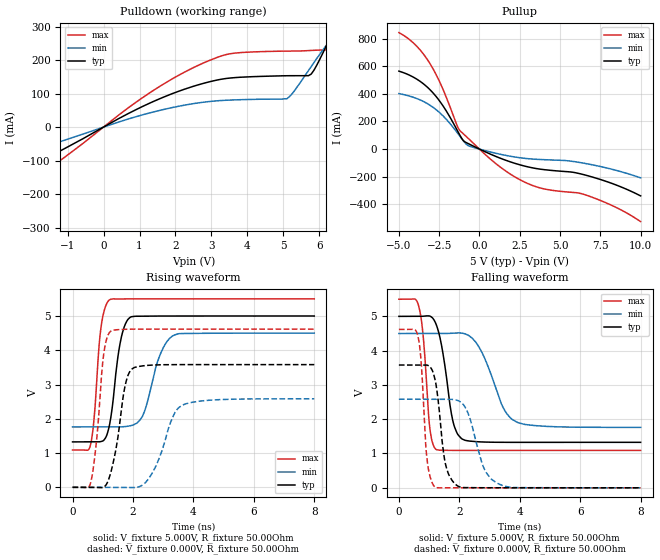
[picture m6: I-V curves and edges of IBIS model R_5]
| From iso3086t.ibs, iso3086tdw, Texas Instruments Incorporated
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|   R_5 MODEL
[Model]   R_5
Model_type   3-state
Polarity   Non-Inverting
Enable   Active-Low
Vmeas   = 2.5V
Vref   = 0V
Cref   = 15pF
|   typ   min   max
|Average C_comp   (Fast PVT)   (Nom PVT)   (Slow PVT)
C_comp   1.85212465pF 1.8517676pF  1.8666174pF
|C_comp (High state)   (Fast PVT)   (Nom PVT)   (Slow PVT)
|C_comp   1.9127669pF  1.9018070pF  1.9152375pF
|C_comp (Low state)   (Fast PVT)   (Nom PVT)   (Slow PVT)
|C_comp   1.7890118pF  1.8017282pF  1.8204679pF
[Model Spec]
Vmeas   2.5V   2.25V   2.75V
[Voltage Range]   5   4.5   5.5
[Temperature Range]   40   125   -40
[Pullup Reference]   5   4.5   5.5
[Pulldown Reference]   0   0   0
[Power Clamp Reference]   5   4.5   5.5
[GND Clamp Reference]   0   0   0
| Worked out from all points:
|   slope of the pulldown table from 0 to 0.75 V, typ, clamps not added: 17.1 ohm
|   slope of the pullup table from 0 to 0.75 V, typ, clamps not added: 18.8 ohm
|   falling waveform, V_fixture 5.000V, R_fixture 50.00Ohm: 20-80 % time 372ps typ, 723ps min, 215ps max; typ from 5 V to 1.33 V
|   rising waveform, V_fixture 5.000V, R_fixture 50.00Ohm: 20-80 % time 316ps typ, 520ps min, 225ps max; typ from 1.33 V to 5 V
|   rising waveform, V_fixture 0.000V, R_fixture 50.00Ohm: 20-80 % time 372ps typ, 626ps min, 264ps max; typ from 0 V to 3.58 V
|   falling waveform, V_fixture 0.000V, R_fixture 50.00Ohm: 20-80 % time 282ps typ, 510ps min, 185ps max; typ from 3.58 V to 0 V
[Pulldown]
|   Voltage   I(typ)   I(min)   I(max)
-5V       -257.1mA   -163.6mA   -354.1mA
-4.246V   -223.8mA   -141.3mA   -309mA
-3.643V   -196mA     -123mA     -271.2mA
-1.683V   -97.4mA    -59.79mA   -136.1mA
1.332V    73.78mA    43.61mA    105.6mA
3.141V    140.1mA    78.28mA    207.2mA
5.101V    153.3mA    84.66mA    226.8mA
5.779V    158.3mA    180.8mA    228.9mA
6.382V    283.1mA    269.4mA    234.2mA
6.457V    299.7mA    279.4mA    249.4mA
6.608V    332.4mA    298.5mA    294.9mA
10V       747mA      509.6mA    1.085A
[Pullup]
|   Voltage   I(typ)   I(min)   I(max)
-5V       564mA      401.4mA    842.8mA
-3.945V   509.9mA    368.1mA    750.4mA
-3.116V   434.9mA    320.6mA    626.6mA
-2.437V   341.9mA    260mA      478.1mA
-1.231V   104.1mA    95.77mA    136.1mA
-1.005V   62.26mA    60.82mA    110.9mA
-703.5mV  40.27mA    25.26mA    78.23mA
1.106V    -57.29mA   -32.6mA    -113.3mA
3.216V    -133.9mA   -71.34mA   -259.6mA
6.683V    -191.4mA   -106.5mA   -335.4mA
8.492V    -260.1mA   -154.1mA   -422.6mA
10V       -338.4mA   -208mA     -524.2mA
[Ramp]
R_load = 50.00Ohm
|   typ   min   max
dV/dt_r   2.148V/372.072ps   1.550V/626.061ps   2.770V/264.463ps
dV/dt_f   2.205V/371.761ps   1.643V/722.711ps   2.646V/214.674ps
[Falling Waveform]
V_fixture = 5.000V
V_fixture_min = 4.500V
V_fixture_max = 5.500V
R_fixture = 50.00Ohm
|   Time   V(typ)   V(min)   V(max)
0s        5V         4.5V       5.5V
670ps     5V         4.5V       5.252V
820ps     5.005V     4.5V       4.27V
1.03ns    5.006V     4.5V       1.696V
1.24ns    4.751V     4.5V       1.113V
1.78ns    1.973V     4.508V     1.09V
2.09ns    1.425V     4.51V      1.09V
2.64ns    1.341V     4.121V     1.09V
3.88ns    1.325V     1.926V     1.09V
8ns       1.326V     1.762V     1.09V
[Rising Waveform]
V_fixture = 5.000V
V_fixture_min = 4.500V
V_fixture_max = 5.500V
R_fixture = 50.00Ohm
|   Time   V(typ)   V(min)   V(max)
0s        1.326V     1.762V     1.09V
590ps     1.325V     1.762V     1.221V
940ps     1.335V     1.761V     4.652V
1.23ns    1.846V     1.76V      5.475V
1.58ns    4.23V      1.763V     5.498V
1.92ns    4.967V     1.798V     5.5V
2.32ns    4.995V     2.084V     5.5V
2.87ns    4.999V     3.808V     5.5V
3.34ns    5V         4.432V     5.5V
8ns       5V         4.5V       5.5V
[Rising Waveform]
V_fixture = 0.000V
V_fixture_min = 0.000V
V_fixture_max = 0.000V
R_fixture = 50.00Ohm
|   Time   V(typ)   V(min)   V(max)
0s        33.95uV    39.73uV    28.54uV
610ps     416.9uV    206.5uV    172.7mV
810ps     -4.552mV   231.9uV    1.495V
1.03ns    1.955mV    335.5uV    3.881V
1.26ns    411.8mV    455.2uV    4.553V
1.74ns    2.965V     -4.456mV   4.612V
2.03ns    3.489V     -9.215mV   4.617V
2.62ns    3.567V     389.7mV    4.618V
3.68ns    3.582V     2.413V     4.618V
8ns       3.581V     2.583V     4.617V
[Falling Waveform]
V_fixture = 0.000V
V_fixture_min = 0.000V
V_fixture_max = 0.000V
R_fixture = 50.00Ohm
|   Time   V(typ)   V(min)   V(max)
0s        3.581V     2.583V     4.617V
630ps     3.581V     2.583V     4.426V
750ps     3.583V     2.583V     3.518V
930ps     3.579V     2.583V     845.6mV
1.21ns    3.101V     2.584V     13.16mV
1.54ns    700.4mV    2.586V     161.5uV
1.97ns    41.06mV    2.54V      -52.37uV
2.84ns    646.9uV    526.3mV    26.13uV
3.31ns    34.98uV    109.7mV    32.25uV
8ns       33.95uV    39.73uV    28.54uV
